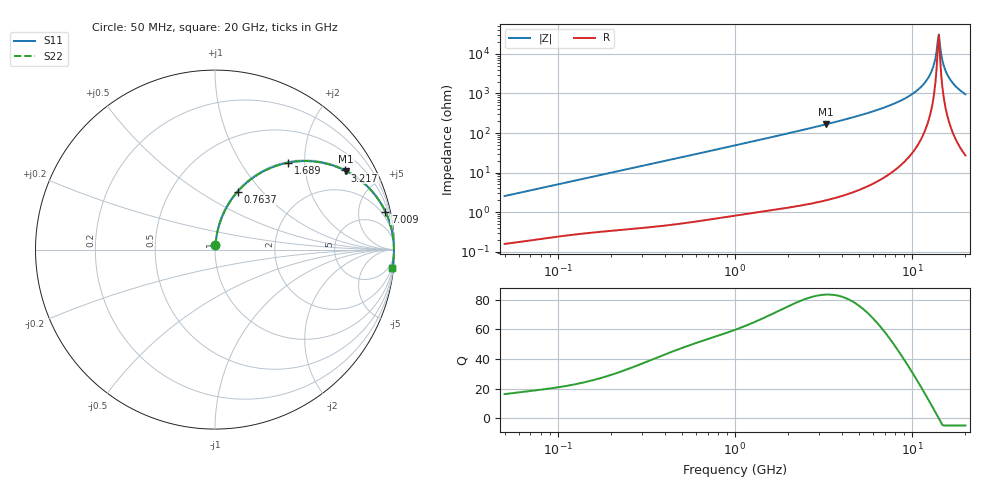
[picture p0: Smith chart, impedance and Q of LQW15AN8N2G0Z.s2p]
!Murata Part Number: LQW15AN8N2G0Z
!These Parameters are Measured in Series Mode Connection
!  o--[Z]--o
!Port1  Port2
!  o-------o
!Freq. Start=50[MHz] Stop=20[GHz], 401[Steps]
# Hz S RI R 50
!Freq.(Hz) S11(Real) S11(Imag) S21(Real) S21(Imag) S12(Real) S12(Imag) S22(Real) S22(Imag)
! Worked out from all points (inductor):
!   401 points, 50 MHz to 20 GHz, reference 50 ohm
!   read as one part in series: L = 8.05 nH near 51.52 MHz
!   highest Q = 83.6 at 3.265 GHz (marker M1), where L = 8.09 nH
!   self-resonance near 13.96 GHz
!   S11 on the Smith chart (normalised r, x): 50 MHz: 1.00, +0.05; 763.7 MHz: 1.01, +0.74; 1.689 GHz: 1.02, +1.65; 3.217 GHz: 1.04, +3.26; 7.009 GHz: 1.15, +8.93; 20 GHz: 2, -19
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5e7  0.00221 0.0253  0.9978 -0.0253  0.9978 -0.0253  0.00221 0.0253
1.364002e8  0.00736 0.067  0.9926 -0.067  0.9926 -0.067  0.00736 0.067
3.721004e8  0.036 0.1747  0.964 -0.1747  0.964 -0.1747  0.036 0.1747
7.636728e8  0.126 0.3229  0.874 -0.3229  0.874 -0.3229  0.126 0.3229
1e9  0.1957 0.3884  0.8043 -0.3884  0.8043 -0.3884  0.1957 0.3884
1.689197e9  0.4073 0.4844  0.5927 -0.4844  0.5927 -0.4844  0.4073 0.4844
2.728004e9  0.6486 0.4714  0.3514 -0.4714  0.3514 -0.4714  0.6486 0.4714
3.216634e9  0.7246 0.4408  0.2754 -0.4408  0.2754 -0.4408  0.7246 0.4408
3.265178e9  0.7311 0.4375  0.2689 -0.4375  0.2689 -0.4375  0.7311 0.4375
7.009217e9  0.949 0.2116  0.051 -0.2116  0.051 -0.2116  0.949 0.2116
7.442007e9  0.9575 0.1928  0.0425 -0.1928  0.0425 -0.1928  0.9575 0.1928
9.745021e9  0.9844 0.1099  0.0156 -0.1099  0.0156 -0.1099  0.9844 0.1099
1.166392e10  0.9936 0.0563  0.00639 -0.0563  0.00639 -0.0563  0.9936 0.0563
1.295331e10  0.9962 0.0255  0.00378 -0.0255  0.00378 -0.0255  0.9962 0.0255
1.334722e10  0.9966 0.0167  0.0034 -0.0167  0.0034 -0.0167  0.9966 0.0167
1.375312e10  0.9968 0.0079  0.00316 -0.0079  0.00316 -0.0079  0.9968 0.0079
1.417136e10  0.9969 -0.000879  0.00309 0.000879  0.00309 0.000879  0.9969 -0.000879
1.438523e10  0.9969 -0.00527  0.00311 0.00527  0.00311 0.00527  0.9969 -0.00527
1.527346e10  0.9964 -0.0228  0.00357 0.0228  0.00357 0.0228  0.9964 -0.0228
1.597544e10  0.9957 -0.036  0.00434 0.036  0.00434 0.036  0.9957 -0.036
1.774144e10  0.9925 -0.067  0.00752 0.067  0.00752 0.067  0.9925 -0.067
2e10  0.9863 -0.1028  0.0137 0.1028  0.0137 0.1028  0.9863 -0.1028
